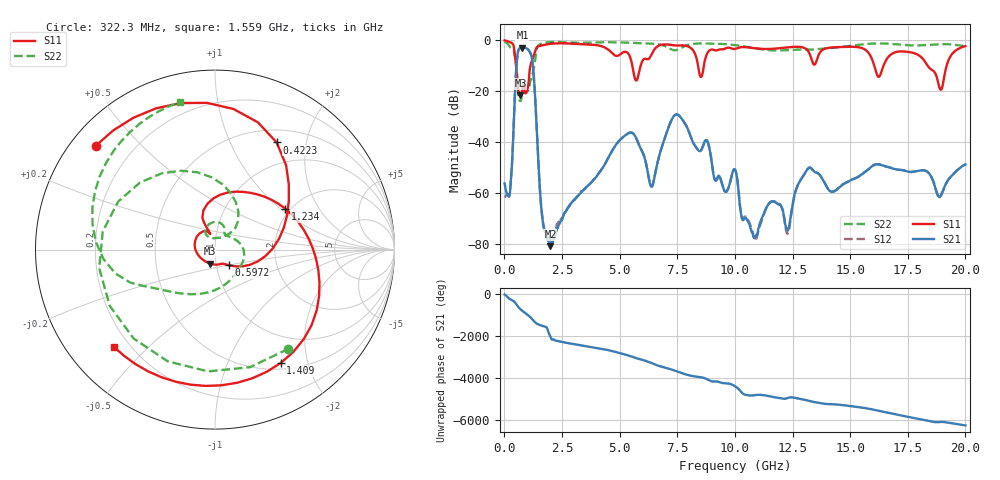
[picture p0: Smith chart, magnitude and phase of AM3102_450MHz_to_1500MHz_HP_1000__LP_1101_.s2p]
!Agilent Technologies,E8364B,MY43040894,A.07.50.67
!Agilent E8364B: A.07.50.67
!Date: Thursday, January 11, 2018 05:59:51
!Correction: S11(Full 2 Port(1,2))
!S21(Full 2 Port(1,2))
!S12(Full 2 Port(1,2))
!S22(Full 2 Port(1,2))
!S2P File: Measurements: S11, S21, S12, S22:
# Hz S  dB  R 50
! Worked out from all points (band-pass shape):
!   1601 points, 10 MHz to 20 GHz, reference 50 ohm
!   highest |S21| = -2.83 dB at 784.6 MHz (marker M1); lowest = -80.9 dB at 1.997 GHz (marker M2)
!   |S21| within 3 dB of the highest: 567.7 MHz to 1.163 GHz (595.2 MHz wide, 68.8 % of centre)
!   lowest |S11| = -21.6 dB at 697.2 MHz (marker M3), VSWR 1.18, Z = 46.9 - j7.42 ohm
!   |S11| at or under -10 dB: 511.4 MHz to 1.128 GHz (616.3 MHz wide, 75.2 % of centre); 16.05 GHz to 16.45 GHz (401.8 MHz wide, 2.47 % of centre); 18.36 GHz to 19.18 GHz (820.6 MHz wide, 4.37 % of centre)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
!   |S22| runs from -23.9 to -0.6 dB; largest |S21 - S12| = 0.0017
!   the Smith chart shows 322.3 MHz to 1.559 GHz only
!   S11 on the Smith chart (normalised r, x): 322.3 MHz: 0.07, +0.37; 422.3 MHz: 0.67, +1.52; 597.2 MHz: 1.14, -0.20; 1.234 GHz: 1.89, +1.08; 1.409 GHz: 0.58, -1.58; 1.559 GHz: 0.14, -0.39
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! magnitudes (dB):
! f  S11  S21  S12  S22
! 10 MHz  -0.1  -56.2  -61.7  -0.6
! 322.3 MHz  -1.1  -50.0  -49.6  -3.3
! 422.3 MHz  -3.2  -28.3  -28.3  -4.4
! 597.2 MHz  -18.8  -4.2  -4.2  -20.5
! 697.2 MHz  -21.6  -2.9  -2.9  -23.9
! 784.6 MHz  -19.2  -2.8  -2.8  -19.0
! 1.234 GHz  -6.9  -9.8  -9.8  -12.8
! 1.409 GHz  -2.7  -36.0  -36.0  -3.1
! 1.559 GHz  -2.1  -61.0  -61.3  -1.5
! 1.997 GHz  -1.4  -80.9  -78.3  -0.7
! 3.346 GHz  -1.5  -59.7  -59.3  -1.0
! 5.395 GHz  -5.5  -36.4  -36.4  -1.0
! 6.682 GHz  -2.2  -46.6  -46.6  -1.6
! 7.494 GHz  -2.0  -29.1  -29.1  -3.8
! 10.01 GHz  -3.4  -50.8  -50.8  -1.9
! 10.89 GHz  -3.1  -77.2  -77.6  -3.1
! 11.62 GHz  -3.3  -63.2  -63.4  -3.9
! 12.3 GHz  -2.7  -74.6  -75.8  -3.8
! 13.34 GHz  -8.0  -50.6  -50.6  -3.7
! 16.68 GHz  -6.3  -49.8  -49.8  -1.3
! 18.93 GHz  -19.4  -61.1  -61.2  -1.5
! 20 GHz  -2.3  -48.8  -48.8  -2.3
